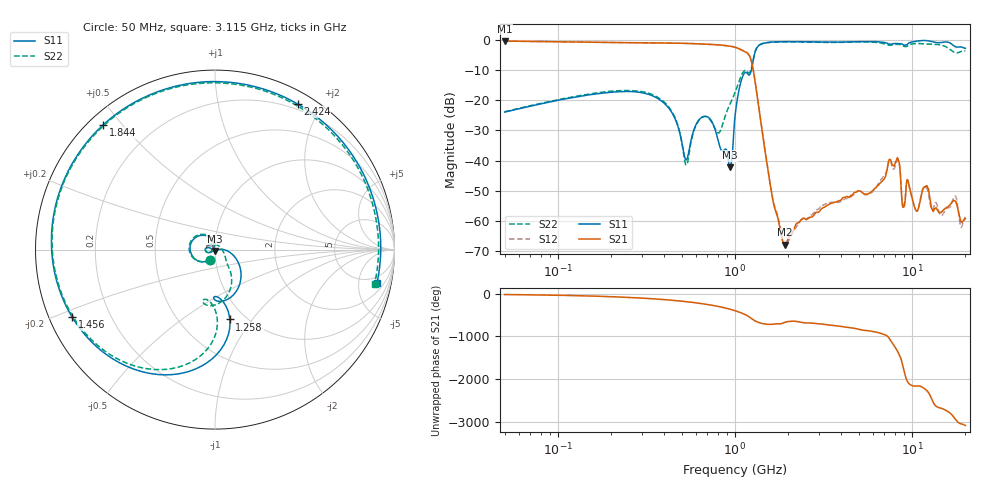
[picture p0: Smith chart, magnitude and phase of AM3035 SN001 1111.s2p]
# Hz S DB R 50
!freq MagS11 AngS11 MagS21 AngS21 MagS12 AngS12 MagS22 AngS22
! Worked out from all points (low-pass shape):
!   1601 points, 50 MHz to 20.05 GHz, reference 50 ohm
!   highest |S21| = -0.39 dB at 50 MHz (marker M1); lowest = -67.9 dB at 1.921 GHz (marker M2)
!   |S21| within 3 dB of the highest: start of sweep to 1.094 GHz
!   lowest |S11| = -42.2 dB at 936 MHz (marker M3), VSWR 1.02, Z = 49.9 - j0.773 ohm
!   |S11| at or under -10 dB: start of sweep to 1.239 GHz
!   |S22| runs from -41.5 to -0.6 dB; largest |S21 - S12| = 0.012
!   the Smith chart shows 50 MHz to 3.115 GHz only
!   S11 on the Smith chart (normalised r, x): 50 MHz: 0.94, -0.11; 1.258 GHz: 0.85, -0.78; 1.456 GHz: 0.07, -0.22; 1.844 GHz: 0.04, +0.45; 2.424 GHz: 0.14, +1.71; 3.115 GHz: 3.37, -8.37
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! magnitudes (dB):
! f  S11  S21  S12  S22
! 50 MHz  -23.9  -0.4  -0.4  -23.8
! 135.9 MHz  -18.6  -0.7  -0.7  -18.4
! 369.6 MHz  -19.6  -1.0  -1.0  -19.2
! 457.6 MHz  -25.9  -1.1  -1.1  -25.7
! 531.6 MHz  -39.8  -1.2  -1.1  -41.5
! 683.3 MHz  -25.3  -1.4  -1.4  -25.4
! 811.8 MHz  -34.3  -1.7  -1.7  -30.8
! 936 MHz  -42.2  -2.1  -2.1  -21.4
! 1.005 GHz  -24.5  -2.4  -2.5  -17.2
! 1.258 GHz  -8.0  -8.8  -8.7  -7.5
! 1.456 GHz  -1.1  -34.1  -33.9  -1.1
! 1.844 GHz  -0.6  -65.8  -64.6  -0.6
! 1.921 GHz  -0.6  -67.9  -68.2  -0.6
! 2.424 GHz  -0.6  -59.1  -59.5  -0.7
! 2.722 GHz  -0.6  -58.7  -58.1  -0.8
! 3.115 GHz  -0.7  -55.8  -54.9  -0.8
! 5.802 GHz  -0.5  -50.7  -51.0  -0.7
! 7.402 GHz  -1.4  -40.0  -40.3  -1.8
! 8.345 GHz  -1.2  -39.5  -39.7  -1.5
! 8.96 GHz  -1.7  -55.5  -54.7  -2.0
! 12.05 GHz  -0.2  -48.5  -48.9  -1.4
! 20.05 GHz  -2.8  -59.3  -58.7  -3.6
